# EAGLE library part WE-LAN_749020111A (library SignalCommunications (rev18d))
WE-LAN LAN Transformer 10/100 Base T - Compliant with IEEE 802.3, IEEE 802.3af and IEEE 802.3at standards - SMT -- Ethernet -- Power over Ethernet -- 1 Gigabit Ethernet -- Compliant with most IC's for ethernet applications like Intel, AMD, Globespan and Realtek -- Hub, Router, Switch Details see: http://katalog.we-online.de/en/pbs/WE-LAN/7490100111A 2016 (C) Würth Elektronik
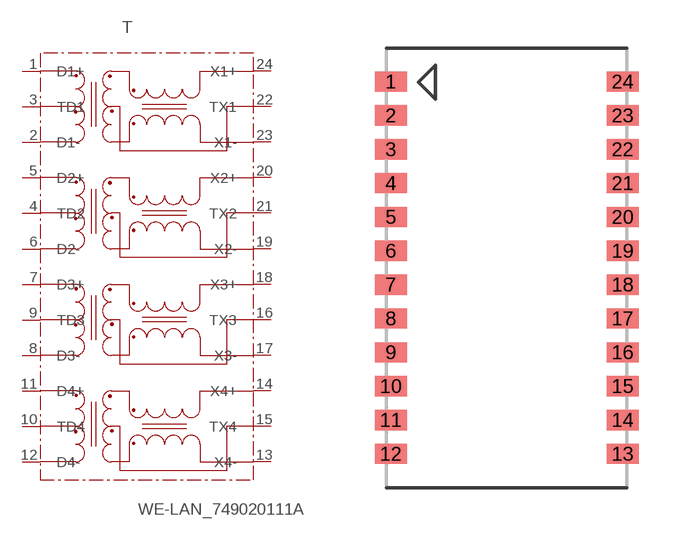
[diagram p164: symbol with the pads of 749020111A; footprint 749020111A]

Designator prefix T

## WE-LAN_749020111A  [749020111A]
1  D1+
2  D1-
3  TD1
4  TD2
5  D2+
6  D2-
7  D3+
8  D3-
9  TD3
10  TD4
11  D4+
12  D4-
13  X4-
14  X4+
15  TX4
16  TX3
17  X3-
18  X3+
19  X2-
20  X2+
21  TX2
22  TX1
23  X1-
24  X1+

## Footprint 749020111A (pad centres in mm)
smd 1.2 x 0.76: 1 -4.35,6.985; 2 -4.35,5.715; 3 -4.35,4.445; 4 -4.35,3.175; 5 -4.35,1.905; 6 -4.35,0.635; 7 -4.35,-0.635; 8 -4.35,-1.905; 9 -4.35,-3.175; 10 -4.35,-4.445; 11 -4.35,-5.715; 12 -4.35,-6.985; 13 4.35,-6.985; 14 4.35,-5.715; 15 4.35,-4.445; 16 4.35,-3.175; 17 4.35,-1.905; 18 4.35,-0.635; 19 4.35,0.635; 20 4.35,1.905; 21 4.35,3.175; 22 4.35,4.445; 23 4.35,5.715; 24 4.35,6.985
